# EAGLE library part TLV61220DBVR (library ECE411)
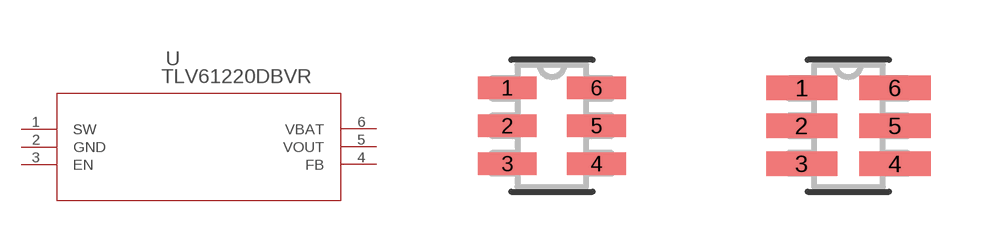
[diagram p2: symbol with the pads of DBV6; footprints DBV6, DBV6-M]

Designator prefix U

## TLV61220DBVR (MANUFACTURER_PART_NUMBER: TLV61220DBVR; VENDOR: Texas Instruments)  [DBV6]
1  SW  in
2  GND  pwr
3  EN  in
4  FB  in
5  VOUT  out
6  VBAT  in

## TLV61220DBVRDBV6-M (MANUFACTURER_PART_NUMBER: TLV61220DBVR; VENDOR: Texas Instruments)  [DBV6-M]
Pads as for DBV6

## TLV61220DBVRDBV6-L (MANUFACTURER_PART_NUMBER: TLV61220DBVR; VENDOR: Texas Instruments)  [DBV6-L]
Pads as for DBV6

## Footprint DBV6 (pad centres in mm)
smd 1.473 x 0.559: 1 -1.118,0.95; 2 -1.118,0; 3 -1.118,-0.95; 4 1.118,-0.95; 5 1.118,0; 6 1.118,0.95

## Footprint DBV6-M (pad centres in mm)
smd 1.778 x 0.61: 1 -1.168,0.95; 2 -1.168,0; 3 -1.168,-0.95; 4 1.168,-0.95; 5 1.168,0; 6 1.168,0.95

## Footprint DBV6-L (pad centres in mm)
smd 1.168 x 0.508: 1 -1.067,0.95; 2 -1.067,0; 3 -1.067,-0.95; 4 1.067,-0.95; 5 1.067,0; 6 1.067,0.95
